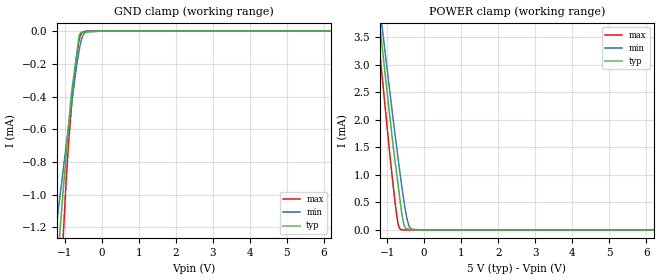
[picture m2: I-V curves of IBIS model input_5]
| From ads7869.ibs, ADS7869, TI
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|   input_5 Model
[Model]   input_5
Model_type   Input
Vinl = 1.5
Vinh = 3.5
|   typ   min   max
|   (nom PVT)   (fast PVT)   (slow PVT)
|C_comp from frequency sweep method (F=16MHz)
|Average
|C_comp   2.246e-12   2.174e-12   2.319e-12
|C_comp from LC tank measurement(L=1nH)
|Average
|Resonant Frequency(Hz)   3.610e+09   3.640e+09   3.570e+09
C_comp   1.946e-12   1.914e-12   1.990e-12
| Where nom  PVT is Nominal Process, 5V, 36C
|   Fast PVT is Strong Process,  5.5V, -40C
|   Slow PVT is Weak Process,   4.5V, 96C
[Model Spec]
|Subparameter   typ   min   max
Vinh   3.5   3.15   3.85
Vinl   1.5   1.35   1.65
[Voltage Range]   5   4.5   5.5
|Ambient Temperature   25   85   -40
|Junction Temperature
[Temperature Range]   36   96   -40
[Power Clamp Reference]   5   4.5   5.5
[GND Clamp Reference]   0   0   0
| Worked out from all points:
|   GND clamp passes 1 mA (typ) near -1.05 V on its own axis
|   POWER clamp passes 1 mA (typ) near -0.74 V on its own axis
[GND Clamp]
|   Voltage   I(typ)   I(min)   I(max)
-5V       -12.82mA   -8.599mA   -23.08mA
-1.247V   -1.57mA    -1.239mA   -2.294mA
-1.123V   -1.215mA   -1.006mA   -1.662mA
-1.029V   -948.8uA   -830.4uA   -1.217mA
-963mV    -767.8uA   -709.6uA   -935.1uA
-902.5mV  -603.7uA   -598.9uA   -717.4uA
-792.5mV  -343.3uA   -411.1uA   -407.7uA
-688mV    -165.7uA   -233.4uA   -174.2uA
-605mV    -24.74uA   -114.5uA   -52.61uA
-560mV    -8.848uA   -65.19uA   -20.54uA
-392mV    -6.194uA   -1.233uA   0A
10V       0A         0A         0A
[POWER Clamp]
|   Voltage   I(typ)   I(min)   I(max)
-5V       28.13mA    26.55mA    30.5mA
-1.25V    4.049mA    4.349mA    3.586mA
-1.036V   2.721mA    3.123mA    2.113mA
-875mV    1.753mA    2.225mA    1.043mA
-748.5mV  1.054mA    1.537mA    303.9uA
-704.5mV  823uA      1.303mA    119.6uA
-638.5mV  476.2uA    966.3uA    8.873uA
-600mV    279.8uA    772.2uA    5.219uA
-540mV    88.21uA    499.5uA    0A
-414.5mV  13.96uA    82.69uA    0A
-239mV    8.05uA     0A         0A
10V       0A         0A         0A
